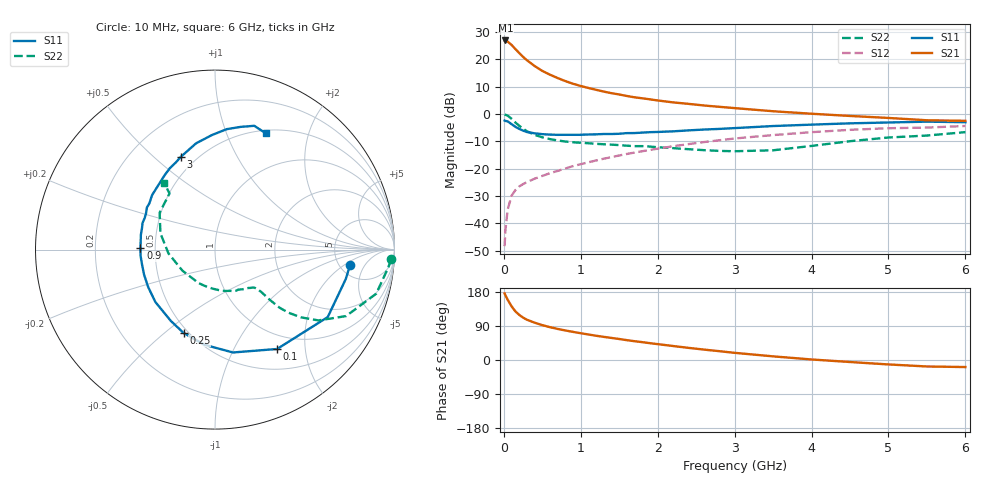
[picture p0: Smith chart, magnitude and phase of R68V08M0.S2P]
! SIEMENS Small Signal Semiconductors
! BFR193
! Si NPN RF Bipolar Junction Transistor in SOT23
! VCE = 8 V  IC = 8 mA
! Common Emitter S-Parameters:  May  1996
# GHz  S  MA  R  50
!  f  S11  S21  S12  S22
! GHz  MAG  ANG  MAG  ANG  MAG  ANG  MAG  ANG
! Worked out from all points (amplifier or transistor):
!   36 points, 10 MHz to 6 GHz, reference 50 ohm
!   highest |S21| = 26.9 dB at 20 MHz (marker M1)
!   |S21| within 3 dB of that: start of sweep to 145.7 MHz
!   unconditionally stable (mu >= 1): 807.2 MHz to 2.034 GHz
!   at 250 MHz: K = 0.56, MSG = 23.3 dB, |S12| = -25.7 dB
!   at 1.4 GHz: K = 1.05, MAG = 10.3 dB, |S12| = -15.8 dB
!   at 6 GHz: K = 0.95, MSG = 0.9 dB, |S12| = -4.4 dB
!   lowest NFmin = 1.25 dB at 450 MHz
!   S11 on the Smith chart (normalised r, x): 10 MHz: 6.18, -2.52; 100 MHz: 0.78, -1.51; 250 MHz: 0.47, -0.58; 900 MHz: 0.41, +0.01; 3 GHz: 0.41, +0.62; 6 GHz: 0.53, +1.39
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0.01  0.7572 -6.6  22.17 175.7  0.0038 87.5  0.9838 -3.1
0.02  0.7468 -12.7  22.18 171.0  0.0074 84.3  0.9684 -6.3
0.05  0.732 -30.9  21.11 159.0  0.0177 74.9  0.9312 -15.3
0.1  0.6529 -58.0  18.39 141.9  0.0318 64.9  0.8188 -26.9
0.15  0.5818 -80.1  15.47 128.3  0.0403 58.5  0.6984 -34.4
0.2  0.5335 -96.3  13.05 119.1  0.047 55.2  0.6085 -38.3
0.25  0.4962 -110.7  11.11 111.8  0.052 53.4  0.5379 -40.7
0.3  0.4674 -121.7  9.647 106.3  0.0565 53.5  0.4833 -42.0
0.4  0.4424 -138.6  7.548 98.5  0.0654 54.3  0.4149 -42.5
0.5  0.427 -150.5  6.144 92.0  0.0734 55.7  0.374 -42.5
0.6  0.4191 -160.6  5.236 86.6  0.0825 57.1  0.3466 -42.5
0.7  0.4149 -168.2  4.545 82.0  0.0908 58.7  0.3276 -42.9
0.9  0.4154 179.0  3.573 74.2  0.1111 60.2  0.303 -44.2
1.1  0.4211 168.8  2.99 67.3  0.1305 61.1  0.2909 -47.2
1.3  0.43 160.0  2.569 61.0  0.152 60.9  0.2788 -50.6
1.6  0.4463 148.2  2.133 52.3  0.1854 60.0  0.2625 -57.7
2.2  0.481 130.2  1.63 36.9  0.2565 55.4  0.2368 -76.5
3  0.5514 110.1  1.281 18.9  0.3555 45.7  0.2079 -116.0
3.5  0.6014 100.1  1.122 9.6  0.411 38.3  0.2163 -147.4
4.5  0.6739 84.5  0.92 -5.3  0.5127 23.2  0.3174 163.4
5.5  0.7236 72.4  0.767 -17.1  0.564 7.3  0.4026 129.0
6  0.7071 66.5  0.749 -18.6  0.6026 2.7  0.4651 127.4
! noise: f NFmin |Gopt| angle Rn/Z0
0.45  1.25  0.23  133  0.12
0.9  1.3  0.35  156  0.11
1.8  2  0.55  -155  0.13
